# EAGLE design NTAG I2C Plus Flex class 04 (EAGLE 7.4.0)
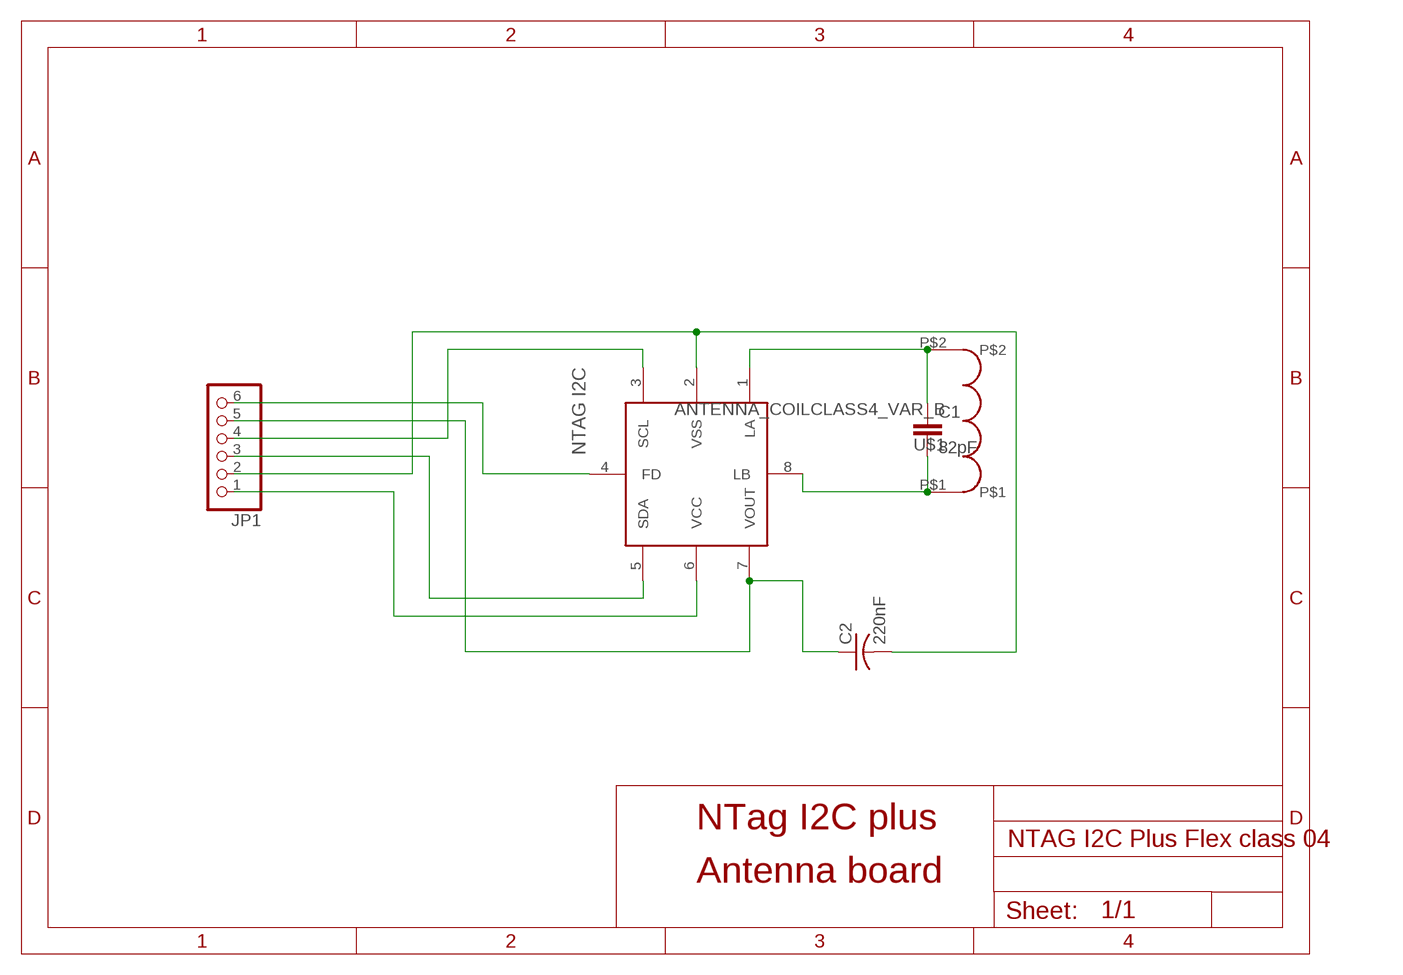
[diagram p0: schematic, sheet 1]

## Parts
C1  82pF  C-EUC0603  [C0603]
C2  220nF  C-USC0805  [C0805]
JP1  PINHD-1X6/90  [1X06/90]
NTAGUI  NTAG_I2C  [XQFN8]
U$1  ANTENNA_COILCLASS4_VAR_B  [L_PICC_50PF_CLASS4_B]

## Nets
+VCC: JP1.1 NTAGUI.6(VCC)
FD: JP1.6 NTAGUI.4(FD)
N$1: C1.1 NTAGUI.1(LA) U$1.P$2
N$2: C1.2 NTAGUI.8(LB) U$1.P$1
SCL: JP1.4 NTAGUI.3(SCL)
SDA: JP1.3 NTAGUI.5(SDA)
VOUT: C2.1 JP1.5 NTAGUI.7(VOUT)
VSS: C2.2 JP1.2 NTAGUI.2(VSS)

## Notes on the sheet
- NTag I2C plus
- Antenna board

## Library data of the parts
C1 = rcl:C-EU: CAPACITOR, European symbol
C2 = rcl:C-US: CAPACITOR, American symbol
JP1 = pinhead (2):PINHD-1X6: PIN HEADER
NTAGUI = NTAG I2C:NTAG_I2C
U$1 = NXP_PICC_Antennas:ANTENNA_COIL: Antenna coils designs for Class 4, Class 5 and Class 6

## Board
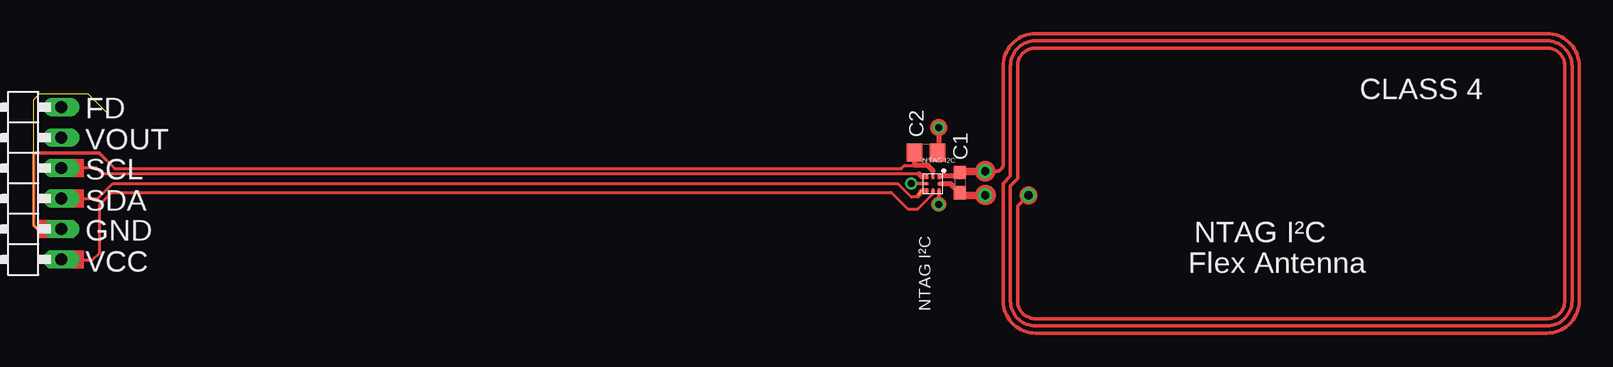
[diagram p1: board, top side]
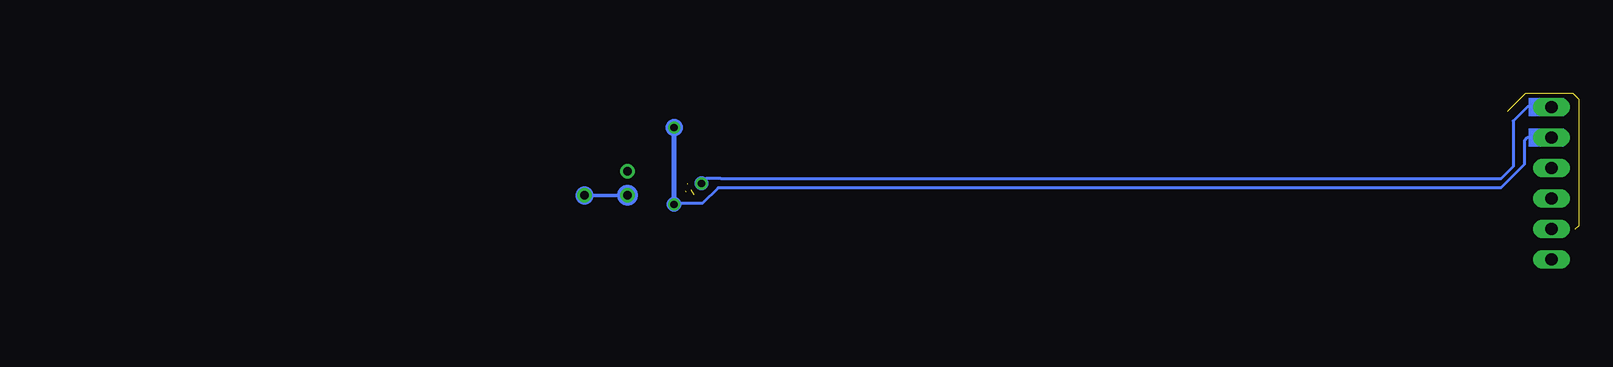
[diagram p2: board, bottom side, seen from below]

No outline drawn. Coordinates in mm, seen from the top.
Copper layers (1*16): Top 0.035mm / dielectric 1.5mm / Bottom 0.035mm
Design rules "default": minimum track width 10mil, minimum drill 24mil, track to track 8mil, track to pad 8mil, pad to pad 8mil, via to via 8mil, smd to smd 8mil, copper to edge 40mil, drill to drill 8mil, minimum pad ring 10mil, minimum via ring 8mil, stop-mask expansion 4mil, vias tented up to drill 0mil, thermal gap 10mil

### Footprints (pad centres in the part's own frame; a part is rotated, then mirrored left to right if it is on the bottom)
C0603 = smd 1.1 x 1: 1 -0.85,0; 2 0.85,0
C0805 = smd 1.3 x 1.5: 1 -0.95,0; 2 0.95,0
1X06/90 = drill 1.016 long: 1 -6.35,-3.81; 2 -3.81,-3.81; 3 -1.27,-3.81; 4 1.27,-3.81; 5 3.81,-3.81; 6 6.35,-3.81
XQFN8 = smd 0.4 x 0.32: 1 -0.6,0.55 | smd 0.4 x 0.22: 2 -0.6,0; 3 -0.6,-0.5; 5 0.6,-0.5; 6 0.6,0; 7 0.6,0.5 | smd 0.22 x 0.4: 4 0,-0.6; 8 0,0.6
L_PICC_50PF_CLASS4_B = drill 0.7: P$1 25.5,1; P$2 25.5,-1; P$3 21.9,1

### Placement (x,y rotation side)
C1  86.09,14.56 270 top
C2  83.26,17.09 180 top
JP1  7.4,14.5 90 top
NTAGUI  83.84,14.46 270 top
U$1  113.7,14.5 180 top

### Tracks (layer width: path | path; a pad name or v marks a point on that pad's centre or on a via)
+VCC
  Top 0.254: JP1.1 11.26,8.1 13.8,8.1 14.4,8.7 14.4,12.72 15.43,13.75 80.36,13.75 81.79,12.33 82.54,12.33 83.84,13.63 83.84,13.64
  Top 0.3: 83.84,13.64 NTAGUI.6
FD  (via drill 0.6)  (1 unrouted)
  Top 0.3: v82.04,14.5 82.75,14.5 83.24,14.5 83.3,14.5
  Bottom 0.254: JP1.6 11.26,20.9 13.2,20.9 14.4,19.7 14.4,15.9 15.4,14.9 80.45,14.91 81.64,14.91 v82.04,14.5
N$1
  Top 0.254: 86.18,15.5 arc90 C1.1
  Top 0.3: NTAGUI.1 86.09,15.06 C1.1
  Top 0.61: U$1.P$2 86.09,15.5 C1.1
N$2
  Top 0.406: C1.2 85.34,14.46 NTAGUI.8
  Top 0.61: U$1.P$1 86.09,13.5 C1.2
N$3
  Top 0.3: 84.35,13.5 84.35,13.9
N$7
  Top 0.3: 82.9,15.15 83.3,15.15 83.3,15 82.9,15
N$8
  Top 0.3: 82.75,13.65 82.5,13.4
N$9
  Top 0.3: 85.85,15.2 84.55,15.2 84.4,15.05 84.4,15.2 84.45,15.2
N$10
  Top 0.3: 83.85,13.75 83.85,13.9
SCL
  Top 0.254: 82.69,15.28 14.64,15.28 14.15,15.77 JP1.4
  Top 0.3: NTAGUI.3 82.91,15.06
  Top 0.406: 82.91,15.06 82.69,15.28
SDA  (2 unrouted)
  Top 0.254: JP1.3 13.47,13.23 13.48,13.22 14.25,13.22 15.51,14.49 80.91,14.49 82.05,13.35 82.61,13.35 82.75,13.49 82.85,13.86
  Top 0.3: 82.9,13.95 83.3,13.95 83.3,13.8 82.85,13.8
  Top 0.406: 82.65,13.51 82.85,13.86
VOUT  (via drill 0.6)
  Top 0.3: v84.34,12.75 NTAGUI.7
  Top 0.406: v84.34,12.75 v84.33,12.75 | v84.33,19.15 84.33,17.09 C2.1
  Bottom 0.254: JP1.5 13.21,18.31 13.47,18.05 13.47,16.08 15.42,14.13 80.66,14.13 81.96,12.83 84.25,12.83 v84.33,12.75
  Bottom 0.406: v84.33,12.75 v84.33,19.15
VSS  (5 unrouted)
  Top 0.254: JP1.2 9.21,10.69 | 82.3,16 81.5,16 81.22,15.72 15.66,15.72 14.9,16.48
  Top 0.3: NTAGUI.2 83.84,15.57 | 14.9,16.48 14.9,16.5 14.35,17.05 9.05,17.05 8.9,16.9 8.9,11 9.2,10.7 | 9.2,10.7 9.21,10.69 | 9.2,10.7 9.75,10.7
  Top 0.406: C2.2 82.31,16.01 82.3,16 83.41,16 83.84,15.57
(copper drawn outside any net)
  shapes: Bottom area x2, Bottom circle x12, Top area x4, Top circle x22

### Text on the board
tNames: CLASS 4 | FD | VOUT | SCL | SDA | GND | NTAG I²C | VCC | Flex Antenna | NTAG I²C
